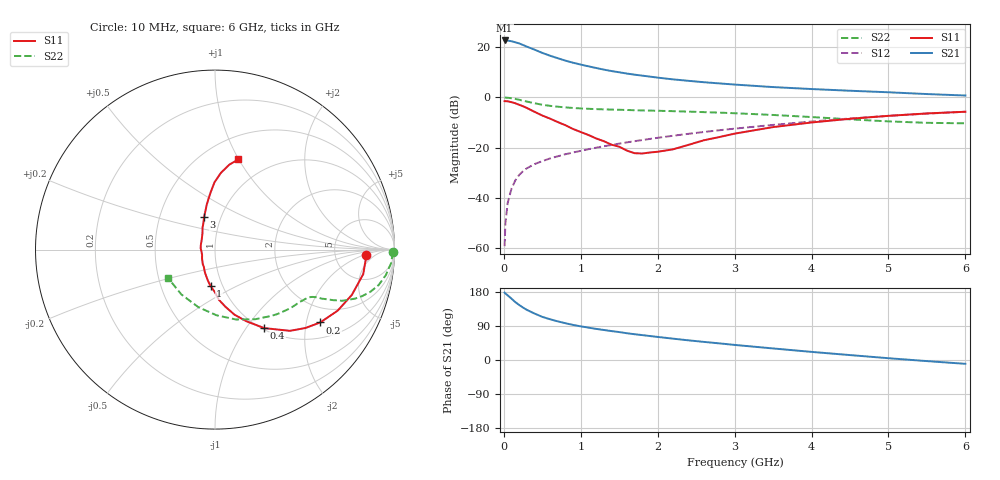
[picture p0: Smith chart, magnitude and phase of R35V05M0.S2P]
! SIEMENS Small Signal Semiconductors
! BFR181
! Si NPN RF Bipolar Junction Transistor in SOT23
! VCE = 5 V  IC = 5 mA
! Common Emitter S-Parameters:  May  1996
# GHz  S  MA  R  50
!  f  S11  S21  S12  S22
! GHz  MAG  ANG  MAG  ANG  MAG  ANG  MAG  ANG
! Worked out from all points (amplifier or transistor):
!   36 points, 10 MHz to 6 GHz, reference 50 ohm
!   highest |S21| = 22.7 dB at 10 MHz (marker M1)
!   |S21| within 3 dB of that: start of sweep to 344.3 MHz
!   unconditionally stable (mu >= 1): 1.16 GHz to 2.992 GHz
!   at 250 MHz: K = 0.42, MSG = 25.1 dB, |S12| = -29.3 dB
!   at 1.4 GHz: K = 1.04, MAG = 13.5 dB, |S12| = -18.9 dB
!   at 6 GHz: K = 0.86, MSG = 3.2 dB, |S12| = -5.7 dB
!   lowest NFmin = 1.55 dB at 450 MHz
!   S11 on the Smith chart (normalised r, x): 10 MHz: 11, -2; 200 MHz: 1.46, -2.42; 400 MHz: 1.02, -1.22; 1 GHz: 0.88, -0.37; 3 GHz: 0.83, +0.31; 6 GHz: 0.72, +0.99
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0.01  0.843 -1.9  13.57 177.8  0.0011 94.3  0.9917 -0.8
0.02  0.8419 -3.6  13.39 175.7  0.0031 87.9  0.989 -1.7
0.05  0.8371 -9.4  13.49 170.6  0.008 84.7  0.9842 -4.4
0.1  0.8033 -18.3  13.09 161.8  0.0154 81.0  0.9624 -8.5
0.15  0.7632 -26.5  12.46 152.6  0.0225 75.6  0.933 -12.2
0.2  0.7131 -34.7  11.85 145.1  0.0288 72.8  0.8971 -15.2
0.25  0.667 -40.9  11.01 138.3  0.0342 68.9  0.859 -17.6
0.3  0.6159 -47.3  10.21 132.2  0.039 68.2  0.8264 -19.3
0.4  0.5163 -57.9  8.899 122.5  0.0472 65.2  0.764 -21.9
0.5  0.4361 -66.3  7.677 113.8  0.0541 63.8  0.7147 -23.2
0.6  0.3788 -73.3  6.756 107.6  0.061 63.4  0.6796 -24.0
0.8  0.2801 -85.6  5.39 97.1  0.0741 63.0  0.6328 -25.0
1  0.2049 -97.0  4.493 88.8  0.0865 64.1  0.6033 -25.9
1.1  0.1789 -102.5  4.151 85.4  0.0934 64.2  0.5935 -26.5
1.3  0.1348 -115.3  3.568 79.2  0.1069 64.4  0.5781 -27.9
1.6  0.0875 -145.6  2.979 70.6  0.1276 64.1  0.5619 -30.6
2.2  0.0928 142.7  2.283 56.3  0.1728 62.4  0.5327 -37.6
3  0.1904 108.6  1.801 39.8  0.2392 57.9  0.4845 -49.7
3.5  0.2568 100.2  1.605 30.5  0.284 53.9  0.4476 -60.1
4.5  0.3755 90.4  1.357 13.0  0.3812 43.9  0.366 -88.7
5.5  0.4803 80.4  1.166 -2.9  0.4761 31.5  0.3123 -126.9
6  0.5186 75.5  1.09 -10.1  0.5197 24.5  0.3051 -148.2
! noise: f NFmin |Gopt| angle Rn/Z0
0.45  1.55  0.48  17  0.36
0.9  1.65  0.4  35  0.34
1.8  2  0.18  88  0.34
